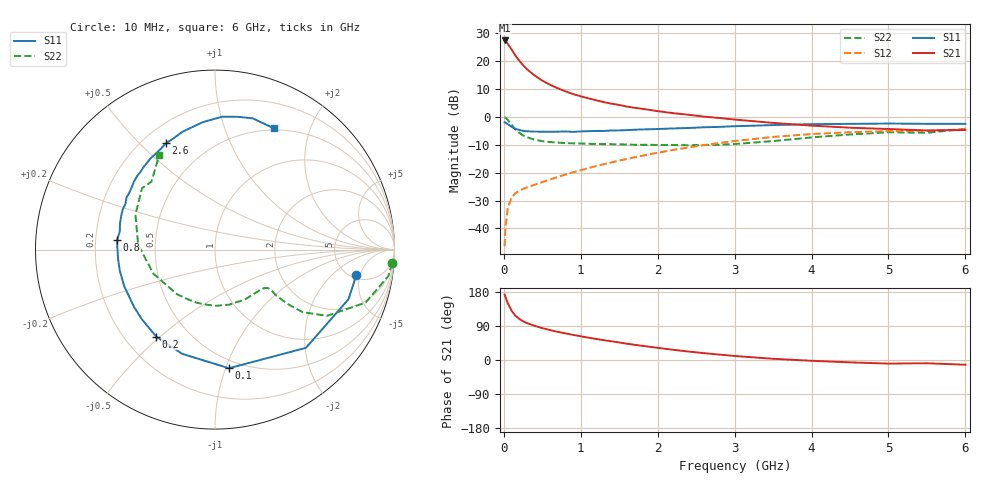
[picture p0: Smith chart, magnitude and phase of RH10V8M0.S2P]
! SIEMENS Small Signal Semiconductors
! BFR106
! Si NPN RF Bipolar Junction Transistor in SOT23
! VCE = 10 V  IC = 8 mA
! Common Emitter S-Parameters:  August  1996
# GHz  S  MA  R  50
!  f  S11  S21  S12  S22
! GHz  MAG  ANG  MAG  ANG  MAG  ANG  MAG  ANG
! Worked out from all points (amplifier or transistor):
!   36 points, 10 MHz to 6 GHz, reference 50 ohm
!   highest |S21| = 27.4 dB at 10 MHz (marker M1)
!   |S21| within 3 dB of that: start of sweep to 94.89 MHz
!   unconditionally stable (mu >= 1): 544.6 MHz to 1.896 GHz; 5.293 GHz to end of sweep
!   at 250 MHz: K = 0.63, MSG = 22.2 dB, |S12| = -25.8 dB
!   at 1.4 GHz: K = 1.10, MAG = 8.6 dB, |S12| = -16.3 dB
!   at 6 GHz: K = 1.01, MAG = -0.6 dB, |S12| = -4.4 dB
!   S11 on the Smith chart (normalised r, x): 10 MHz: 5.52, -4.35; 100 MHz: 0.43, -1.03; 200 MHz: 0.33, -0.49; 800 MHz: 0.29, +0.04; 2.6 GHz: 0.29, +0.60; 6 GHz: 0.48, +1.49
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0.01  0.8004 -10.2  23.55 172.7  0.0048 83.7  0.9892 -4.4
0.02  0.7934 -20.4  23.1 167.2  0.0099 79.8  0.9772 -8.7
0.05  0.7459 -47.2  20.6 150.0  0.0227 68.3  0.8894 -19.4
0.1  0.6655 -83.3  16.28 130.4  0.036 55.2  0.7252 -30.6
0.15  0.6087 -107.6  12.63 116.9  0.0428 47.9  0.6 -35.5
0.2  0.585 -124.0  10.23 108.6  0.0472 45.6  0.5216 -36.6
0.25  0.5627 -136.4  8.455 102.0  0.051 45.7  0.4648 -36.9
0.3  0.5524 -144.9  7.183 97.5  0.0545 46.6  0.4321 -36.9
0.4  0.5456 -158.1  5.542 90.2  0.0606 48.8  0.3898 -36.0
0.5  0.5434 -167.5  4.475 84.1  0.0677 52.1  0.367 -35.9
0.6  0.5425 -174.6  3.781 79.0  0.0755 54.6  0.3551 -37.0
0.8  0.5481 174.5  2.879 70.3  0.0925 58.9  0.3396 -40.2
0.9  0.54 169.3  2.573 66.3  0.1015 60.3  0.3361 -42.0
1.1  0.5553 160.2  2.155 59.0  0.1209 62.5  0.3297 -47.6
1.3  0.5605 152.9  1.845 52.3  0.1422 63.5  0.3249 -53.4
1.6  0.5798 143.1  1.533 43.0  0.176 63.7  0.3198 -63.7
2.2  0.6216 125.5  1.169 27.0  0.2555 59.8  0.3132 -88.6
2.6  0.6521 114.7  1.015 18.1  0.3115 55.0  0.3128 -108.9
3.5  0.7136 95.4  0.782 3.2  0.4378 40.6  0.3685 -158.6
4.5  0.751 80.1  0.641 -6.2  0.5308 22.0  0.484 156.4
5.5  0.7522 68.2  0.572 -8.6  0.5631 9.3  0.5185 133.1
6  0.7512 64.2  0.583 -12.5  0.6003 1.2  0.6123 120.4
